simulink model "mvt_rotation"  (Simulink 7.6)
settings: Solver=ode15s  StartTime=0.0  StopTime=2  RelTol=1e-3
libraries: fl_lib x6, nesl_utility x4

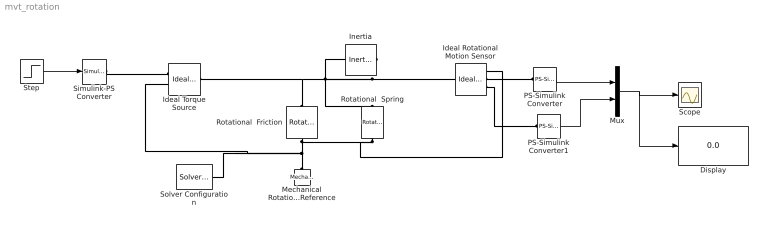
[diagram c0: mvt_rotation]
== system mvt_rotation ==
  Display : Display
  Ideal Rotational Motion Sensor : fl_lib/Mechanical/Mechanical Sensors/Ideal Rotational Motion Sensor  DialogController=NetworkEngine.DynNeDlgSource  SystemSampleTime=-1  offset=0 rad  w_Log=off  t_Log=off  phi_Log=off  LocalVarNames=|w|t|phi  LocalVarDescs=|w|t|phi  LocalVarLogging=[0 0 0]
  Ideal Torque Source : fl_lib/Mechanical/Mechanical Sources/Ideal Torque Source  DialogController=NetworkEngine.DynNeDlgSource  SystemSampleTime=-1  w_Log=off  t_Log=off  LocalVarNames=|w|t  LocalVarDescs=|w|t  LocalVarLogging=[0 0]
  Inertia : fl_lib/Mechanical/Rotational Elements/Inertia  DialogController=NetworkEngine.DynNeDlgSource  SystemSampleTime=-1  inertia=0.01 kg*m^2  initial_velocity=0 rad/s  t_Log=off  LocalVarNames=|t  LocalVarDescs=|t  LocalVarLogging=0
  Mechanical Rotational Reference : fl_lib/Mechanical/Rotational Elements/Mechanical Rotational Reference  DialogController=NetworkEngine.DynNeDlgSource  SystemSampleTime=-1  t_Log=off  LocalVarNames=|t  LocalVarDescs=|t  LocalVarLogging=0
  Mux : Mux  Inputs=2
  PS-Simulink Converter : nesl_utility/PS-Simulink Converter  DialogController=NetworkEngine.DynNeUtilDlgSource  SystemSampleTime=-1  PhysicalDomain=network_engine_domain  LeftPortType=input  RightPortType=output  SubClassName=ps_output  Unit=1  AffineConversion=off
  PS-Simulink Converter1 : nesl_utility/PS-Simulink Converter  DialogController=NetworkEngine.DynNeUtilDlgSource  SystemSampleTime=-1  PhysicalDomain=network_engine_domain  LeftPortType=input  RightPortType=output  SubClassName=ps_output  Unit=1  AffineConversion=off
  Rotational  Spring : fl_lib/Mechanical/Rotational Elements/Rotational Spring  DialogController=NetworkEngine.DynNeDlgSource  SystemSampleTime=-1  spr_rate=10 N*m/rad  init_def=0 rad  t_Log=off  w_Log=off  phi_Log=off  LocalVarNames=|t|w|phi  LocalVarDescs=|t|w|phi  LocalVarLogging=[0 0 0]
  Rotational  Friction : fl_lib/Mechanical/Rotational Elements/Rotational Friction  DialogController=NetworkEngine.DynNeDlgSource  SystemSampleTime=-1  brkwy_trq=0.001 N*m  Col_trq=0.00001 N*m  visc_coef=0.1 N*m/(rad/s)  trans_coef=10 s/rad  vel_thr=1e-4 rad/s  t_Log=off  w_Log=off  LocalVarNames=|t|w  LocalVarDescs=|t|w  LocalVarLogging=[0 0]
  Scope : Scope
  Simulink-PS Converter : nesl_utility/Simulink-PS Converter  DialogController=NetworkEngine.DynNeUtilDlgSource  SystemSampleTime=-1  PhysicalDomain=network_engine_domain  LeftPortType=input  RightPortType=output  SubClassName=ps_input  Unit=1  AffineConversion=off  InputFilterTimeConstant=.001  UdotUserProvided=0
  Solver Configuration : nesl_utility/Solver Configuration  DialogController=NetworkEngine.DynNeUtilDlgSource  SystemSampleTime=-1  PhysicalDomain=network_engine_domain  LeftPortType=input  RightPortType=generic  SubClassName=solver  Accelerate=off  Profile=off  ResidualTolerance=1e-9  MaxNonlinIter=3  MaxModeIter=2  DoFixedCost=off  UseLocalSampling=off  DoDC=off  LinearAlgebra=Sparse  LocalSolverSampleTime=.001  LocalSolverChoice=NE_BACKWARD_EULER_ADVANCER  UseLocalSolver=off
  Step : Step  Time=0.2  After=1000  SampleTime=0
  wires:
  Step/1 -> Simulink-PS Converter/1
  PS-Simulink Converter/1 -> Mux/1
  PS-Simulink Converter1/1 -> Mux/2
  Mux/1 -> Scope/1, Display/1
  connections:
  Rotational  Spring/RConn1 -- Rotational  Friction/RConn1 -- Mechanical Rotational Reference/LConn1 -- Ideal Torque Source/RConn2 -- Solver Configuration/RConn1 -- Ideal Rotational Motion Sensor/RConn1
  Ideal Rotational Motion Sensor/LConn1 -- Rotational  Spring/LConn1 -- Ideal Torque Source/LConn1 -- Rotational  Friction/LConn1 -- Inertia/LConn1
  Simulink-PS Converter/RConn1 -- Ideal Torque Source/RConn1
  Ideal Rotational Motion Sensor/RConn2 -- PS-Simulink Converter/LConn1
  Ideal Rotational Motion Sensor/RConn3 -- PS-Simulink Converter1/LConn1
